| TEXAS INSTRUMENTS INCORPORATED
| Digital Light Processing Group
| IBIS Model of DLP6500_TypeA
| P65_1080P
| This device can be powered at the following Vccs:
|  3.3 volt Vcc
| This file provides unique models under the [Model Selector] for each Vcc.
| For operation at a specific Vcc, select the appropriate model after each
| [Model Selector] keyword.
[IBIS Ver]   3.2
[Comment char]  |_char
[File Name]   dlp6500_type_a.ibs
[File Rev]   0.0 | f_die
[Date]   December 23, 2011
[Source]   Data created from TI-SPICE simulations at TI-DLP.
[Notes]   The following is an IBIS list for the P65_1080P.
[Disclaimer] Property of Texas Instruments Incorporated.  Unauthorized
   reproduction and/or distribution is strictly prohibited.
   This product is protected under copyright law.
   Created  2011, (C) Copyright  2011, Texas Instruments
   Incorporated, All Rights Reserved
   UNLESS THERE IS A SIGNED, WRITTEN AGREEMENT TO THE
   CONTRARY, TEXAS INSTRUMENTS (TI) IS PROVIDING THE IBIS
   MODELS  AND WITHOUT ANY WARRANTY, EXPRESSED OR
   IMPLIED.  TI assumes no liability for:
   1) the accuracy of the IBIS models provided to your
   company;
   2) the proper functioning of these IBIS Models in your
   design or for any resulting applications; or
   3) infringement of patents, copyrights or intellectual
   property rights resulting from your use of these IBIS
   models.
   TI provides IBIS Models as a service to our customers.
   You and your company shall not distribute, sell or give
   these models to anyone else without prior written
   permission from TI.
   TI reserves the right to make changes to our products or
   to discontinue any semiconductor product or service
   without notice, and advises our customers to obtain the
   latest version of relevant information to verify, before
   placing orders, that the information being relied on is
   current.
   Please be aware that your receipt and use of the IBIS
   information provided shall serve as acceptance of these
   terms and conditions.  If you do not accept these terms,
   you should return or destroy the IBIS models and any
   other accompanying information immediately.
| Component P65_1080P_PW 203-pin Device
[Component]   P65_1080P_PW
[Manufacturer]   Texas Instruments, Inc.
[Package]
|   typ   min   max
R_pkg   2.64e+00   5.11e-01   3.62e+00
L_pkg   3.31e-09   1.16e-09   6.57e-09
C_pkg   4.45e-12   2.38e-12   8.80e-12
|MBRESET PINS SHOULD BE TIED TO A 250pF CAPACITOR TO GROUND
[Pin]   signal_name   model_name   R_pin   L_pin   C_pin
A1   VSS   GND
A3   VRESET   POWER
A5   VRESET   POWER
A7   VCC   POWER
A9   VSS   GND
A11   D_AP(1)   INPUT_LVDS_BUF   2.82E+00   1.26E-09   3.53E-12
A13   D_AN(1)   INPUT_LVDS_BUF   2.84E+00   1.26E-09   3.54E-12
A15   VCC   POWER
A17   D_AN(5)   INPUT_LVDS_BUF   2.82E+00   1.26E-09   3.52E-12
A19   D_AP(5)   INPUT_LVDS_BUF   2.83E+00   1.26E-09   3.53E-12
A21   VCCI   POWER
A23   D_AP(6)   INPUT_LVDS_BUF   2.83E+00   1.26E-09   3.53E-12
A25   D_AN(6)   INPUT_LVDS_BUF   2.83E+00   1.26E-09   3.53E-12
A27   VCCI   POWER
A29   D_AP(8)   INPUT_LVDS_BUF   2.82E+00   2.28E-09   3.86E-12
B2   SCPDO   OUTPUT_BUF   1.60E+00   1.94E-09   3.80E-12
B4   VRESET   POWER
B6   RESERVED_STM   NC
B8   VSS   GND
B10   D_AN(0)   INPUT_LVDS_BUF   2.83E+00   2.10E-09   3.81E-12
B12   D_AP(0)   INPUT_LVDS_BUF   2.82E+00   2.10E-09   3.81E-12
B14   VSS   GND
B16   D_AP(4)   INPUT_LVDS_BUF   2.82E+00   2.72E-09   4.02E-12
B18   D_AN(4)   INPUT_LVDS_BUF   2.82E+00   2.73E-09   4.01E-12
B20   VSS   GND
B22   DCLK_AN   INPUT_LVDS_BUF   2.82E+00   1.96E-09   3.76E-12
B24   DCLK_AP   INPUT_LVDS_BUF   2.82E+00   1.96E-09   3.76E-12
B26   VSS   GND
B28   D_AP(9)   INPUT_LVDS_BUF   2.82E+00   3.37E-09   4.23E-12
B30   VSS   GND
C1   VCC   POWER
C3   PWRDNZ   INPUT_BUF   1.19E+00   2.87E-09   3.37E-12
C5   RESET_A(0)   INPUT_BUF   3.32E+00   2.87E-09   7.44E-12
C7   VRESET   POWER
C9   RESERVED_BB   NC
C11   RESET_MODE(1)   INPUT_BUF   2.41E+00   3.54E-09   5.95E-12
C13   VSS   GND
C15   D_AP(3)   INPUT_LVDS_BUF   2.82E+00   3.72E-09   4.35E-12
C17   D_AN(3)   INPUT_LVDS_BUF   2.82E+00   3.75E-09   4.35E-12
C19   VSS   GND
C21   SCTRL_AN   INPUT_LVDS_BUF   2.82E+00   3.75E-09   4.35E-12
C23   SCTRL_AP   INPUT_LVDS_BUF   2.82E+00   3.73E-09   4.35E-12
C25   VSS   GND
C27   D_AP(10)   INPUT_LVDS_BUF   2.83E+00   4.12E-09   4.48E-12
C29   D_AN(8)   INPUT_LVDS_BUF   2.83E+00   2.27E-09   3.87E-12
D2   RESERVED_XI1   NC
D4   SCPENZ   INPUT_BUF   1.41E+00   3.71E-09   4.11E-12
D6   VSS   GND
D8   RESET_MODE(0)   INPUT_BUF   3.09E+00   6.57E-09   8.39E-12
D10   RESERVED_TS   NC
D12   EN_BIAS   OUTPUT_BUF   5.11E-01   3.72E-09   2.38E-12
D14   D_AP(2)   INPUT_LVDS_BUF   2.83E+00   3.78E-09   4.37E-12
D16   D_AN(2)   INPUT_LVDS_BUF   2.83E+00   3.72E-09   4.35E-12
D18   VSS   GND
D20   D_AP(7)   INPUT_LVDS_BUF   2.82E+00   5.01E-09   4.77E-12
D22   D_AN(7)   INPUT_LVDS_BUF   2.82E+00   5.04E-09   4.79E-12
D24   VSS   GND
D26   D_AP(11)   INPUT_LVDS_BUF   2.82E+00   5.13E-09   4.82E-12
D28   D_AN(9)   INPUT_LVDS_BUF   2.82E+00   3.38E-09   4.23E-12
D30   VCCI   POWER
E1   VCC   POWER
E3   SCPCLK   INPUT_BUF   1.23E+00   2.71E-09   3.38E-12
E5   RESET_A(1)   INPUT_BUF   2.98E+00   4.42E-09   7.39E-12
E27   D_AN(10)   INPUT_LVDS_BUF   2.82E+00   4.12E-09   4.48E-12
E29   VSS   GND
F2   VSS   GND
F4   SCPDI   INPUT_BUF   1.55E+00   3.63E-09   4.35E-12
F26   D_AN(11)   INPUT_LVDS_BUF   2.83E+00   5.13E-09   4.82E-12
F28   VSS   GND
F30   D_AP(12)   INPUT_LVDS_BUF   2.83E+00   2.16E-09   3.83E-12
G1   VOFFSET   POWER
G3   RESETZ   INPUT_BUF   2.87E+00   2.71E-09   6.52E-12
G5   RESET_A(2)   INPUT_BUF   2.74E+00   4.42E-09   6.93E-12
G27   VSS   GND
G29   D_AN(12)   INPUT_LVDS_BUF   2.82E+00   2.15E-09   3.82E-12
H2   EN_RESET   OUTPUT_BUF   1.73E+00   1.94E-09   4.04E-12
H4   VSS   GND
H6   NO_CONNECT   NC
H26   VSS   GND
H28   D_AN(13)   INPUT_LVDS_BUF   2.83E+00   3.58E-09   4.30E-12
H30   D_AP(13)   INPUT_LVDS_BUF   2.83E+00   3.59E-09   4.31E-12
J1   VOFFSET   POWER
J3   VSS   GND
J5   MBRST<13>   NC
J25   VSS   GND
J27   D_AN(14)   INPUT_LVDS_BUF   2.84E+00   3.95E-09   4.44E-12
J29   D_AP(14)   INPUT_LVDS_BUF   2.83E+00   3.92E-09   4.42E-12
K2   VSS   GND
K4   MBRST<9>   NC
K6   MBRST<14>   NC
K26   D_AN(15)   INPUT_LVDS_BUF   2.83E+00   5.42E-09   4.91E-12
K28   D_AP(15)   INPUT_LVDS_BUF   2.82E+00   5.45E-09   4.92E-12
K30   VSS   GND
L1   VOFFSET   POWER
L3   MBRST<7>   NC
L5   MBRST<10>   NC
L25   VSS   GND
L27   VSS   GND
L29   VSS   GND
M2   VSS   GND
M4   MBRST<4>   NC
M6   VSS   GND
M26   VSS   GND
M28   VSS   GND
M30   VCCI   POWER
N1   VOFFSET   POWER
N3   MBRST<3>   NC
N5   VBIAS   POWER
N25   VSS   GND
N27   D_BN(15)   INPUT_LVDS_BUF   2.82E+00   5.27E-09   4.86E-12
N29   VSS   GND
P2   MBRST<0>   NC
P4   VBIAS   POWER
P6   RESERVED_TP1   NC
P26   D_BP(15)   INPUT_LVDS_BUF   2.83E+00   5.24E-09   4.86E-12
P28   D_BP(14)   INPUT_LVDS_BUF   2.82E+00   4.91E-09   4.74E-12
P30   VSS   GND
R1   VOFFSET   POWER
R3   VBIAS   POWER
R5   VBIAS   POWER
R25   VSS   GND
R27   D_BN(14)   INPUT_LVDS_BUF   2.82E+00   4.85E-09   4.72E-12
R29   D_BN(13)   INPUT_LVDS_BUF   2.83E+00   3.26E-09   4.20E-12
T2   VSS   GND
T4   RESET_SEL(0)   INPUT_BUF   1.64E+00   3.76E-09   4.57E-12
T6   RESET_IRQZ   OUTPUT_BUF   1.23E+00   5.23E-09   4.33E-12
T26   VSS   GND
T28   D_BP(13)   INPUT_LVDS_BUF   2.83E+00   3.26E-09   4.20E-12
T30   D_BN(12)   INPUT_LVDS_BUF   2.82E+00   2.13E-09   3.82E-12
U1   VCC   POWER
U3   RESERVED_BA   NC
U5   RESET_SEL(1)   INPUT_BUF   1.22E+00   4.77E-09   4.14E-12
U27   VSS   GND
U29   D_BP(12)   INPUT_LVDS_BUF   2.82E+00   2.26E-09   3.86E-12
V2   RESET_STROBE   INPUT_BUF   1.36E+00   2.02E-09   3.37E-12
V4   PG_RESET   INPUT_BUF   3.62E+00   4.95E-09   8.80E-12
V26   D_BN(11)   INPUT_LVDS_BUF   2.82E+00   5.10E-09   4.81E-12
V28   VSS   GND
V30   VSS   GND
W1   RESET_OEZ   INPUT_BUF   1.57E+00   1.16E-09   3.44E-12
W3   RESERVED_TP2   NC
W5   VSS   GND
W27   D_BN(10)   INPUT_LVDS_BUF   2.83E+00   4.12E-09   4.48E-12
W29   VSS   GND
Y2   RESERVED_TP0   NC
Y4   VSS   GND
Y6   MBRST<8>   NC
Y8   MBRST<12>   NC
Y10   PG_OFFSET   INPUT_BUF   2.51E+00   5.92E-09   7.03E-12
Y12   VSS   GND
Y14   D_BP(2)   INPUT_LVDS_BUF   2.77E+00   4.39E-09   4.51E-12
Y16   D_BN(2)   INPUT_LVDS_BUF   2.77E+00   4.43E-09   4.52E-12
Y18   VSS   GND
Y20   D_BP(7)   INPUT_LVDS_BUF   2.76E+00   4.86E-09   4.65E-12
Y22   D_BN(7)   INPUT_LVDS_BUF   2.76E+00   4.85E-09   4.66E-12
Y24   VSS   GND
Y26   D_BP(11)   INPUT_LVDS_BUF   2.82E+00   5.13E-09   4.82E-12
Y28   D_BN(9)   INPUT_LVDS_BUF   2.82E+00   3.38E-09   4.23E-12
Y30   VCCI   POWER
AA1   RESERVED_PFE   NC
AA3   VSS   GND
AA5   MBRST<6>   NC
AA7   MBRST<2>   NC
AA9   VSS   GND
AA11   PG_BIAS   INPUT_BUF   2.62E+00   3.50E-09   6.34E-12
AA13   VSS   GND
AA15   D_BP(3)   INPUT_LVDS_BUF   2.82E+00   3.78E-09   4.37E-12
AA17   D_BN(3)   INPUT_LVDS_BUF   2.82E+00   3.79E-09   4.37E-12
AA19   VSS   GND
AA21   SCTRL_BN   INPUT_LVDS_BUF   2.82E+00   3.74E-09   4.35E-12
AA23   SCTRL_BP   INPUT_LVDS_BUF   2.82E+00   3.72E-09   4.34E-12
AA25   VSS   GND
AA27   D_BP(10)   INPUT_LVDS_BUF   2.82E+00   4.12E-09   4.48E-12
AA29   D_BN(8   INPUT_LVDS_BUF   2.82E+00   2.40E-09   3.91E-12
AB2   VCC   POWER
AB4   MBRST<1>   NC
AB6   MBRST<5>   NC
AB8   EN_OFFSET   OUTPUT_BUF   2.93E+00   2.00E-09   6.37E-12
AB10   D_BN(0)   INPUT_LVDS_BUF   2.81E+00   2.98E-09   4.08E-12
AB12   D_BP(0)   INPUT_LVDS_BUF   2.80E+00   2.97E-09   4.08E-12
AB14   VSS   GND
AB16   D_BP(4)   INPUT_LVDS_BUF   2.82E+00   4.40E-09   4.57E-12
AB18   D_BN(4)   INPUT_LVDS_BUF   2.83E+00   4.40E-09   4.58E-12
AB20   VSS   GND
AB22   DCLK_BN   INPUT_LVDS_BUF   2.82E+00   2.10E-09   3.80E-12
AB24   DCLK_BP   INPUT_LVDS_BUF   2.82E+00   2.10E-09   3.80E-12
AB26   VSS   GND
AB28   D_BP(9)   INPUT_LVDS_BUF   2.83E+00   3.37E-09   4.23E-12
AB30   VSS   GND
AC3   RESET_A(3)   INPUT_BUF   2.01E+00   1.16E-09   4.29E-12
AC5   MBRST<11>   NC
AC7   MBRST<15>   NC
AC9   VCC   POWER
AC11   D_BP(1)   INPUT_LVDS_BUF   2.83E+00   1.26E-09   3.53E-12
AC13   D_BN(1)   INPUT_LVDS_BUF   2.83E+00   1.26E-09   3.53E-12
AC15   VCC   POWER
AC17   D_BN(5)   INPUT_LVDS_BUF   2.78E+00   1.26E-09   3.48E-12
AC19   D_BP(5)   INPUT_LVDS_BUF   2.78E+00   1.26E-09   3.48E-12
AC21   VCCI   POWER
AC23   D_BP(6)   INPUT_LVDS_BUF   2.83E+00   1.26E-09   3.53E-12
AC25   D_BN(6)   INPUT_LVDS_BUF   2.83E+00   1.26E-09   3.54E-12
AC27   VCCI   POWER
AC29   D_BP(8)   INPUT_LVDS_BUF   2.82E+00   2.39E-09   3.90E-12
| Model INPUT_LVDS_BUF
[Model Selector]   INPUT_LVDS_BUF
INPUT_LVDS_BUF_33   3.3 volt Vcc
| Model INPUT_BUF
[Model Selector]   INPUT_BUF
INPUT_BUF_33   3.3 volt Vcc
| Model OUTPUT_BUF
[Model Selector]   OUTPUT_BUF
OUTPUT_BUF_33   3.3 volt Vcc
| Models and submodels in the file (3): INPUT_LVDS_BUF_33 (Input), INPUT_BUF_33 (Input), OUTPUT_BUF_33 (Output)
